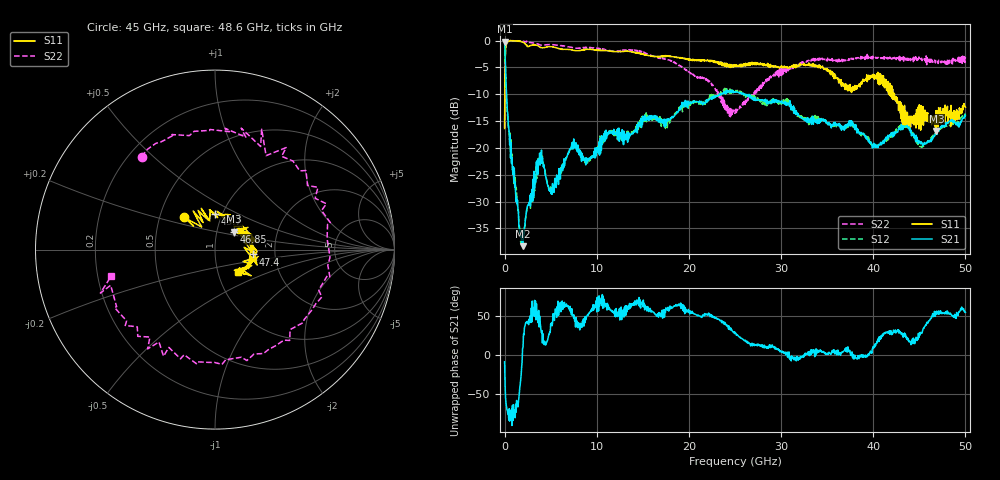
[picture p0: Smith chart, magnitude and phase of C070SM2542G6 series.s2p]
! 7/15/2021 9:06:43 AM
! Y:\C070SM2542G6 SERIES\C070SM2542G6 SERIES.S2P
! CHANNEL.1
! TR.MEASUREMENT
! CORRECTED.DATA
# GHZ S RI R 50.0
! FREQ.GHZ  S11RE  S11IM  S21RE  S21IM  S12RE  S12IM  S22RE  S22IM
!; PortSelection: Port_12
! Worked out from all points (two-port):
!   1001 points, 10 MHz to 50 GHz, reference 50 ohm
!   highest |S21| = -0.18 dB at 10 MHz (marker M1); lowest = -38.3 dB at 1.96 GHz (marker M2)
!   |S21| within 3 dB of the highest: start of sweep to 68.41 MHz
!   lowest |S11| = -16.8 dB at 46.85 GHz (marker M3), VSWR 1.34, Z = 60.2 + j12.3 ohm
!   |S11| at or under -10 dB: start of sweep to 35.87 MHz; 41.74874 GHz to 41.75453 GHz (5.789 MHz wide, 0.0139 % of centre); 42.31 GHz to end of sweep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
!   |S22| runs from -16.3 to 0.0 dB; largest |S21 - S12| = 0.053
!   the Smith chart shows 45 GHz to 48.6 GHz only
!   S11 on the Smith chart (normalised r, x): 45 GHz: 0.66, +0.26; 45.7 GHz: 0.93, +0.38; 46.85 GHz: 1.20, +0.25; 47.4 GHz: 1.54, -0.09; 48.6 GHz: 1.25, -0.32
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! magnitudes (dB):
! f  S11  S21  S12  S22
! 10 MHz  -16.4  -0.2  -0.2  -16.3
! 359.9 MHz  -0.2  -13.7  -14.3  -0.2
! 1.61 GHz  -0.2  -34.6  -34.9  -0.1
! 1.96 GHz  -0.3  -38.3  -38.0  -0.2
! 3.909 GHz  -1.2  -21.0  -20.9  -0.8
! 5.109 GHz  -1.2  -28.2  -27.9  -0.8
! 7.259 GHz  -1.8  -19.8  -20.2  -1.3
! 8.358 GHz  -1.8  -22.5  -22.2  -1.4
! 16.71 GHz  -2.9  -15.2  -14.8  -3.2
! 22.01 GHz  -3.8  -11.4  -11.2  -7.6
! 25 GHz  -4.8  -9.6  -9.5  -13.6
! 33.35 GHz  -4.8  -14.4  -14.1  -3.7
! 37.5 GHz  -8.2  -16.0  -15.6  -3.5
! 40.15 GHz  -7.2  -19.6  -19.5  -3.3
! 41.7 GHz  -8.0  -17.7  -18.3  -3.2
! 43.65 GHz  -15.7  -16.1  -15.6  -3.4
! 45 GHz  -12.0  -18.7  -19.6  -3.6
! 45.7 GHz  -14.0  -19.2  -19.3  -4.0
! 46.85 GHz  -16.8  -17.1  -17.1  -3.9
! 47.4 GHz  -13.4  -15.9  -16.3  -3.8
! 48.6 GHz  -15.0  -14.8  -15.7  -4.5
! 50 GHz  -12.4  -13.9  -13.8  -3.1
